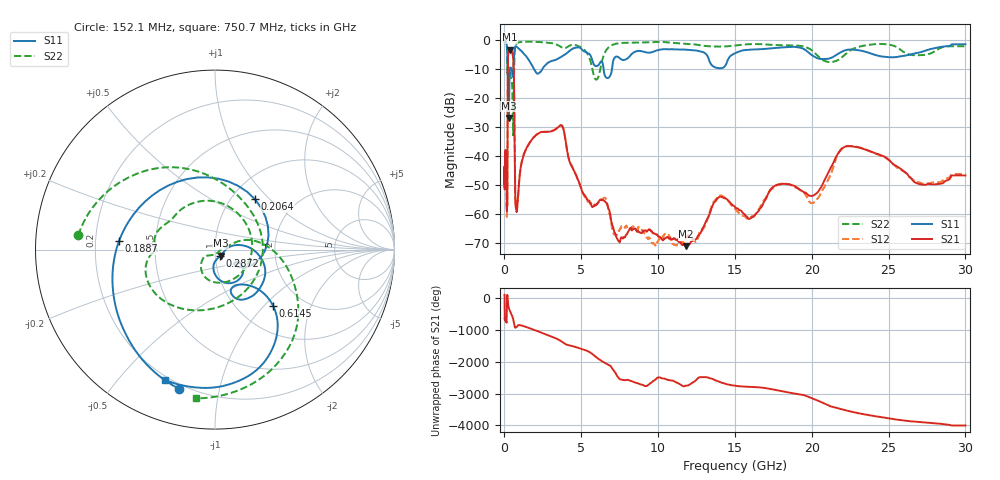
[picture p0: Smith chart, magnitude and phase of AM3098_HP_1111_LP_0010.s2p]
! Date/Time: Thu, Feb 28, 2019 8:47 AM
! Network Analyzer: Agilent Technologies E8364B Rev: A.07.50.67
! Sweep from 0.010 to 30.000 GHz, 1601 Points, Sweep Type: LOG
! Power Supply: 5.022 V, 0.002 A
# Hz S DB R 50
!freq MagS11 AngS11 MagS21 AngS21 MagS12 AngS12 MagS22 AngS22
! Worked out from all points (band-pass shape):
!   1601 points, 10 MHz to 30 GHz, reference 50 ohm
!   highest |S21| = -3.36 dB at 337.1 MHz (marker M1); lowest = -71.1 dB at 11.83 GHz (marker M2)
!   |S21| within 3 dB of the highest: 228.1 MHz to 568 MHz (339.9 MHz wide, 85.4 % of centre)
!   lowest |S11| = -26.9 dB at 288.7 MHz (marker M3), VSWR 1.09, Z = 53.1 - j3.51 ohm
!   |S11| at or under -10 dB: 210 MHz to 367.9 MHz (157.8 MHz wide, 54.6 % of centre); 1.909 GHz to 2.474 GHz (565.7 MHz wide, 25.8 % of centre); 6.45 GHz to 7.002 GHz (552 MHz wide, 8.21 % of centre)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
!   |S22| runs from -32.9 to -0.5 dB; largest |S21 - S12| = 0.012
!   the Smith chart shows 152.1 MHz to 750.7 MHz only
!   S11 on the Smith chart (normalised r, x): 152.1 MHz: 0.18, -0.76; 188.7 MHz: 0.30, +0.04; 206.4 MHz: 1.28, +0.82; 287.2 MHz: 1.05, -0.08; 614.5 MHz: 1.44, -1.12; 750.7 MHz: 0.18, -0.67
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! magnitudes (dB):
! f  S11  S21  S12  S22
! 10 MHz  -0.4  -43.9  -45.5  -0.5
! 38.04 MHz  -0.2  -41.1  -41.0  -0.5
! 97.46 MHz  -0.8  -38.9  -39.7  -1.2
! 144.7 MHz  -1.6  -54.8  -53.6  -2.0
! 152.1 MHz  -1.9  -56.0  -59.4  -2.3
! 188.7 MHz  -5.4  -53.1  -53.2  -9.2
! 206.4 MHz  -8.9  -21.8  -21.8  -8.9
! 227 MHz  -17.5  -6.6  -6.6  -9.4
! 287.2 MHz  -26.8  -3.6  -3.5  -10.2
! 288.7 MHz  -26.9  -3.6  -3.5  -10.2
! 337.1 MHz  -11.9  -3.4  -3.4  -10.7
! 550.5 MHz  -12.8  -5.5  -5.5  -30.9
! 614.5 MHz  -7.0  -12.6  -12.5  -14.7
! 750.7 MHz  -2.2  -57.8  -56.7  -1.6
! 2.084 GHz  -11.5  -32.7  -32.7  -0.7
! 3.723 GHz  -5.8  -29.5  -29.5  -2.6
! 5.989 GHz  -9.1  -56.8  -56.8  -13.7
! 7.926 GHz  -6.7  -67.1  -64.0  -1.0
! 11.83 GHz  -3.4  -71.1  -67.8  -1.4
! 20.2 GHz  -5.9  -53.3  -55.8  -4.6
! 22.56 GHz  -3.4  -36.7  -36.6  -3.5
! 30 GHz  -1.5  -46.7  -46.3  -2.2
